(* Logix 5000 Rung export; software revision 16.04 *)

MODULES
   Local : vendor None type None code None
   MVI69E_AFC : vendor None type None code None
END_MODULES

TYPE AFCEMeterLinearLiquidArchive :   // Different Liquid Archive
STRUCT
   Write : AFCEMeterLinearLiquidArchiveWrite;
   Fetch : AFCEMeterLinearLiquidArchiveFetch;
END_STRUCT
END_TYPE

TYPE AFCESiteAlarms :   // Indicates if a meter has any alarms
STRUCT
   Meter1 : BOOL;   // Meter in alarm
   Meter2 : BOOL;   // Meter in alarm
   Meter3 : BOOL;   // Meter in alarm
   Meter4 : BOOL;   // Meter in alarm
   Meter5 : BOOL;   // Meter in alarm
   Meter6 : BOOL;   // Meter in alarm
   Meter7 : BOOL;   // Meter in alarm
   Meter8 : BOOL;   // Meter in alarm
   Meter9 : BOOL;   // Meter in alarm
   Meter10 : BOOL;   // Meter in alarm
   Meter11 : BOOL;   // Meter in alarm
   Meter12 : BOOL;   // Meter in alarm
   Meter13 : BOOL;   // Meter in alarm
   Meter14 : BOOL;   // Meter in alarm
   Meter15 : BOOL;   // Meter in alarm
   Meter16 : BOOL;   // Meter in alarm
END_STRUCT
END_TYPE

TYPE AFCEMeterLinearLiquid :   // Linear Liquid Meter
STRUCT
   Control : AFCEMeterControl;   // Meter Control
   Status : AFCEMeterStatus;   // Meter Status
   ProcessVariables : AFCEMeterLinearLiquidProcess;   // Input process variables to be transferred to the module
   Analysis : AFCEMeterAnalysis;   // Molar Analysis data to be transferred to the module (only for gas products with online gas chromatograph applications)
   Alarm : AFCEMeterLinearLiquidAlarm;   // Meter Alarms
   Archive : AFCEMeterLinearLiquidArchive;   // Archive
   Profile : AFCEMeterProfile;   // Module profile (meter type/product group) transfered from the module
   Calibration : AFCEMeterLinearLiquidCal;   // Calibration
   BackPlaneReturn : AFCEMeterLinearLiqBackPlaneReturn;
END_STRUCT
END_TYPE

TYPE AFCEFlag :   // Flags contains status information updated by ladder and also trigger bits for clock update
STRUCT
   AFCStopped : BOOL;   // Indicates that the module has sent a new input block to be processed by ladder - UPDATED BY LADDER
   AFCInputSequenceNum : INT;   // Meter number (0 -15) associated to blocks 1-16. Used to update "Profile" (meter type and product group.) UPDATED BY LADDER
END_STRUCT
END_TYPE

TYPE AFCEUtilBlockNonInterrupt :
STRUCT
   Now : BOOL;
   ModbusMasterCommand : BOOL;
   ModbusMasterResponse : BOOL;
   Archive : DINT;
   Prover : BOOL;
   PassThru : BOOL;
   Calibration : BOOL;
END_STRUCT
END_TYPE

TYPE AFCEMeterCalRequestActionType :
STRUCT
   ZeroShift : BOOL;   // Zero Shift
   SetZero : BOOL;   // Set Zero
   SetSpan : BOOL;   // Set Span
   SetMid1 : BOOL;   // Set Mid 1
   SetMid2 : BOOL;   // Set Mid 2
   SetMid3 : BOOL;   // Set Mid 3
END_STRUCT
END_TYPE

TYPE AFCEProveConfigEnable :   // Prove controls at enable
STRUCT
   MeterNumber : INT;   // Meter number requested (1-16)
   AutoAcceptProve : BOOL;   // Auto-accept the prove
   AutoContinueProve : BOOL;   // Auto-continue the prove
END_STRUCT
END_TYPE

TYPE AFCEModbusGateway :   // Modbus Gateway
STRUCT
   Command : AFCEModbusGatewayCommand[10];   // Modbus gateway commands - contains setup and modbus data
END_STRUCT
END_TYPE

TYPE AFCEMeterCalRequestActionValue :
STRUCT
   ZeroShift : AFCEMeterCalRequestValue;   // Zero Shift
   SetZero : AFCEMeterCalRequestValue;   // Set Zero
   SetSpan : AFCEMeterCalRequestValue;   // Set Span
   SetMid1 : AFCEMeterCalRequestValue;   // Set Mid 1
   SetMid2 : AFCEMeterCalRequestValue;   // Set Mid 2
   SetMid3 : AFCEMeterCalRequestValue;   // Set Mid 3
END_STRUCT
END_TYPE

TYPE AFCEMeterLinearLiqBackPlaneReturn :   // Linear Liquid Meter
STRUCT
   StandardDefault : AFCEMeterLinearLiquidStandardDataDflt;
   StandardRaw : INT[14];
   Extended : AFCEExtended;
END_STRUCT
END_TYPE

TYPE AFCEMeterLinearLiquidArchiveDflt :   // Default Configuration
STRUCT
   ClosingTimestamp : DINT;   // Closing Timestamp
   CumulativeActiveStreams : INT;
   CurrentActiveStream : SINT;
   MeterStatus : SINT;
   FlowingPeriod : DINT;
   PeriodDuration : DINT;
   AccumulatorTotalizer : DINT;
   AccumulatorResidue : REAL;
   MeterAlarms : DINT;
   PulseFrequency : REAL;
   Temperature : REAL;
   Pressure : REAL;
   Density : REAL;
   WaterContent : REAL;
   ReferenceDensity : REAL;
   Ctpl : REAL;
   KFactor : REAL;
   MeterFactor : REAL;
   InputPulseCount : DINT;
   ManPulseCountCurrent : DINT;
   MassNRAccumulatorCurrent : REAL;   // Non-resettable
   MassNRAccumulatorOpening : REAL;   // Non-resettable
   Available01 : INT;
   Available02 : INT;
   Available03 : INT;
   Available04 : INT;
   NetNRAccumulatorCurrent : REAL;   // Non-resettable
   NetNRAccumulatorOpening : REAL;   // Non-resettable
   GrossNRAccumulatorCurrent : REAL;   // Non-resettable
   GrossNRAccumulatorOpening : REAL;   // Non-resettable
   GrossStandardNRAccumulatorOpening : REAL;   // Non-resettable
   GrossStandardNRAccumulatorCurrent : REAL;   // Non-resettable
   WaterNRAccumulatorCurrent : REAL;   // Non-resettable
   WaterNRAccumulatorOpening : REAL;   // Non-resettable
   API2540VaporPressureAbsolute : REAL;   // Non-resettable
   Available05 : INT;
   Available06 : INT;
   UserSpecifiedFlowAverage1 : REAL;
   UserSpecifiedFlowAverage2 : REAL;
   UserSpecifiedFlowAverage3 : REAL;
END_STRUCT
END_TYPE

TYPE AFCEMeterAnalysisError :
STRUCT
   StreamOutOfRange : BOOL;   // Requested Stream Number Out of Range
   StreamNotConfigured : BOOL;   // Requested Stream Not Configured
END_STRUCT
END_TYPE

TYPE AFCEMeterLinearLiquidCalRequest :
STRUCT
   ProcessVariable : AFCEMeterLinearLiquidCalRequestProces;   // Process Variable
   ActionType : AFCEMeterCalRequestActionType;   // Action Type
   Value : AFCEMeterCalRequestActionValue;   // Value
   Count : DINT;   // Number of calibration requests
END_STRUCT
END_TYPE

TYPE AFCEMeterCalRequestValue :
STRUCT
   Applied : REAL;   // Applied
   Measured : REAL;   // Measured
END_STRUCT
END_TYPE

TYPE AFCEMeterLinearLiquidStandardDataDflt :   // EAFC Backplane Return Standard Data
STRUCT
   Meter_Alarms : DINT;   // Meter alarms
   NR_Acc_Net_Totalizer : DINT;   // Non-resettable accumulator, net, totalizer (m3)
   NR_Acc_Net_Residue : REAL;   // Non-resettable accumulator, net, residue (m3)
   FlowRate_Net : REAL;   // Flow rate, net (m3/h)
   NR_Acc_Gross_Totalizer : DINT;   // Non-resettable accumulator, gross / indicated, totalizer (m3)
   NR_Acc_GrossStandard_Totalizer : DINT;   // Non-resettable accumulator, gross standard, totalizer (m3)
   NR_Acc_Mass_Totalizer : DINT;   // Non-resettable accumulator, mass, totalizer (kg)
END_STRUCT
END_TYPE

TYPE AFCEModbusMasterDataType :   // Modbus master data type
STRUCT
   Bit : BOOL;   // bit type
   Word : BOOL;   // word type (16-bit)
   Long : BOOL;   // long integer (32-bit)
   LongRemote : BOOL;   // long integer (32-bit)
END_STRUCT
END_TYPE

TYPE AFCEUtil :   // Used for internal ladder logic usage. These values must not be changed by user application.
STRUCT
   Flags : AFCEFlag;   // Wallclock update commands
   CycleCounter : INT;   // Reflects current block ID calculated by ladder to be sent to the module
   Buffer : AFCEUtilBuffer;
   Block : AFCEUtilBlock;
END_STRUCT
END_TYPE

TYPE AFCEWallclock :
STRUCT
   GetAFCTime : BOOL;   // Get current AFC Time
   SetAFCTimeFromPLCTime : BOOL;   // Set AFC time from PLC time. Updates current AFC time
   EnableLocalDateTime : BOOL;   // Enable Local Date Time.
   AFCTime : AFCETime;   // Coordinated Universal Time. Updated by either getting or setting AFC time.
END_STRUCT
END_TYPE

TYPE AFCEProvePhaseBitmap :   // AFC prove phase bitmap
STRUCT
   NotSelected : BOOL;   // Not selected
   Active : BOOL;   // Active, not counting
   CountingPast1stSwitch : BOOL;   // Counting past 1st switch for Udir and forward leg for Bdir)
   Past2ndSwitchFwdLeg : BOOL;   // Past 2nd switch forward leg (bidirectional only)
   Past1stSwithRetLeg : BOOL;   // Past 1st switch return leg (bidirectional only)
   RunComplete : BOOL;   // Run complete. past 2nd switch.
END_STRUCT
END_TYPE

TYPE AFCEMeterLinearLiquidCalRequestProces :
STRUCT
   PulseFrequency : BOOL;   // Pulse Frequency
   Temperature : BOOL;   // Temperature
   Pressure : BOOL;   // Pressure
   Density : BOOL;   // Density
   WaterContent : BOOL;   // Water Content
END_STRUCT
END_TYPE

TYPE AFCEProveInputConfig :   // Prove input block results - prover configuration
STRUCT
   Type : INT;   // Prover type
   Options : INT;   // Prover options
   RunsPerProveTotal : INT;   // Total runs per prove
   RunsPerProveSelected : INT;   // Selected runs per prove
   MaxRunsBeforeAbort : INT;   // Max total runs before abort
   ShortPassesPerRun : INT;   // Short passes per run if bidir = 2 , else 0
END_STRUCT
END_TYPE

TYPE AFCEMeterCalResponse :
STRUCT
   Trigger : BOOL;   // Send Error Code and Values to module to be recorded
   ErrorCode : SINT;   // Error Code to send. 0-4 allowed. 0=No error. 1-4=User defined.
   Value : AFCEMeterCalRequestValue;   // Value to Send
   Count : DINT;   // Number of calibration responses
END_STRUCT
END_TYPE

TYPE AFCEMeterArchiveFetchError :
STRUCT
   ArchiveSelectionInvalid : BOOL;   // Archive File Selection Invalid
   AgeOutsideSize : BOOL;   // Age Outside Configured File Size
   ArchiveNeverWritten : BOOL;   // Age OK but Archive Record Never Written (new or reconfigured meter)
   Reserverd1 : BOOL;
   Reserverd2 : BOOL;
   Reserverd3 : BOOL;
   Reserverd4 : BOOL;
   Reserverd5 : BOOL;
   Reserverd6 : BOOL;
   Reserverd7 : BOOL;
   Reserverd8 : BOOL;
   Reserverd9 : BOOL;
   Reserverd10 : BOOL;
   Reserverd11 : BOOL;
   Reserverd12 : BOOL;
   Reserverd13 : BOOL;
END_STRUCT
END_TYPE

TYPE AFCEModbusGatewayCommand :   // Modbus Gateway Command
STRUCT
   Config : AFCEModbusGatewayConfig;   // Config data to be entered by the user.
   Trigger : BOOL;   // Trigger the Command, when cleared module has responded.
   Data : INT[200];   // Contains modbus data written to the module (write commands)
END_STRUCT
END_TYPE

TYPE AFCEProveConfigAccept :   // Prove controls at accept. If auto-accept is selected must be available at enable
STRUCT
   RequestedInterpolationPoint : INT;   // Requested interpolation point (0 nearest)
   ApplyMFChangeAllStreams : BOOL;   // Apply change in meter factor to all streams
   ApplyMFChangeCurve : BOOL;   // Apply change in meter factor to all curve points
   ApplyNewMF : BOOL;   // CApply new meter factor
END_STRUCT
END_TYPE

TYPE AFCEModbusMasterCommand :   // Modbus Master Command
STRUCT
   Config : AFCEModbusMasterConfig;   // Modbus Master Configuration
   ErrorCode : INT;   // Error Code associated to Modbus Master Command
   Pending : BOOL;   // Pending Modbus Master Command - waiting for Modbus Response
   ReturnedTransactionID : DINT;   // Changes to Config.TransactionID value when response has returned.
   Data : INT[100];   // Read or Write Data
END_STRUCT
END_TYPE

TYPE AFCEMeterStatusMeter :   // Meter Status
STRUCT
   Enabled : BOOL;   // Meter Enable Status, 1=enabled
   EnableAlarm : BOOL;   // If set either: 1. The meter is not configured. 2. The event log is full, the action was not performed.
END_STRUCT
END_TYPE

TYPE AFCEMeterLinearLiquidAlarmControl :   // Linear Liquid Process Alarms
STRUCT
   PulseFrequency : AFCEMeterProcessAlarm;   // Pulse Frequency Alarms
   Temperature : AFCEMeterProcessAlarm;   // Temperature Alarms
   Pressure : AFCEMeterProcessAlarm;   // Pressure Alarms
   Density : AFCEMeterProcessAlarm;   // Density Alarms
   WaterPercent : AFCEMeterProcessAlarm;   // Water Percent Alarms
   MeterPulses : AFCEMeterProcessAlarmFidelity;   // Meter Pulses Alarms
END_STRUCT
END_TYPE

TYPE AFCEMeterControl :   // Enable/Disable Meter and Streams
STRUCT
   Meter : AFCEMeterControlMeter;   // Control the Meter
   Stream : AFCEMeterControlStream;   // Control the Meter Streams
   ResetAccumulators : AFCEMeterSignals;   // Resets for meter accumulators
END_STRUCT
END_TYPE

TYPE AFCEProveSequencing :   // AFC prove sequencing tag for phase selection and ball positioning
STRUCT
   Phase : AFCEProvePhaseBitmap;   // AFC phase sequencing
   BallPositionReady : BOOL;   // Ball position: Ready (Udir & Bdir only; fwd leg Bdir)
   BallPositionSealed : BOOL;   // Ball position: Sealed (Udir & Bdir only; fwd leg Bdir)
   BallPositionReadyBwdLeg : BOOL;   // Ball position: Ready bwd leg (Bdir only)
   BallPositionSealedBwdLeg : BOOL;   // Ball position: Sealed bwd leg (Bdir only)
END_STRUCT
END_TYPE

TYPE AFCEMeterLinearLiquidProcess :   // Linear Liquid Process Variables
STRUCT
   PulseFrequency : REAL;   // Pulse frequency (Hz)
   Temperature : REAL;   // Temperature
   Pressure : REAL;   // Pressure
   Density : REAL;   // Density
   WaterPercent : REAL;   // Water (%)
   MeterPulses : DINT;   // Meter pulses
END_STRUCT
END_TYPE

TYPE AFCEUtilBlockInterrupt :
STRUCT
   Now : BOOL;
   ModbusGateway : DINT;
   EnableDisable : BOOL;
   Analysis : DINT;
END_STRUCT
END_TYPE

TYPE AFCEMeterLinearLiquidCal :   // Processor Mediated Calibration
STRUCT
   Request : AFCEMeterLinearLiquidCalRequest;   // Calibration Request from module
   Response : AFCEMeterCalResponse;   // Processor Response
END_STRUCT
END_TYPE

TYPE AFCEComponents :   // High precision gas component analysis (only supported version 2.07.000)
STRUCT
   C1 : REAL;   // Methane
   N2 : REAL;   // Nitrogen
   CO2 : REAL;   // Carbon Dioxide
   C2 : REAL;   // Ethane
   C3 : REAL;   // Propane
   H20 : REAL;   // Water
   H2S : REAL;   // Hydrogen Sulphide
   H2 : REAL;   // Hydrogen
   CO : REAL;   // Carbon Monoxide
   O2 : REAL;   // Oxygen
   IC4 : REAL;   // Iso-butane
   NC4 : REAL;   // Normal Butane
   IC5 : REAL;   // Iso-pentane
   NC5 : REAL;   // Normal-pentane
   C6 : REAL;   // Hexane
   C7 : REAL;   // Heptane
   C8 : REAL;   // Octane
   C9 : REAL;   // Nonane
   C10 : REAL;   // Decane
   He : REAL;   // Helium
   Ar : REAL;   // Argon
   NeoC5 : REAL;   // Not Used
   UxUser1 : REAL;   // Not Used
   UyUser2 : REAL;   // Not Used
   UxUser3 : REAL;   // Not Used
   UyUser4 : REAL;   // Not Used
   UxUser5 : REAL;   // Not Used
   UyUser6 : REAL;   // Not Used
   UxUser7 : REAL;   // Not Used
   UyUser8 : REAL;   // Not Used
   UxUser9 : REAL;   // Not Used
   UyUser10 : REAL;   // Not Used
END_STRUCT
END_TYPE

TYPE AFCEMeterStatus :   // Status
STRUCT
   Meter : AFCEMeterStatusMeter;   // Meter Status
   Stream : AFCEMeterStatusStream;   // Stream Status
END_STRUCT
END_TYPE

TYPE AFCEUtilBlock :
STRUCT
   ProcessInput : INT;
   InterruptPending : AFCEUtilBlockInterrupt;
   InterruptComplete : AFCEUtilBlockInterrupt;
   NonInterruptPending : AFCEUtilBlockNonInterrupt;
   NonInterruptComplete : AFCEUtilBlockNonInterrupt;
END_STRUCT
END_TYPE

TYPE AFCEModbusGatewayConfig :   // Modbus Ggateway Configuration
STRUCT
   Enable : BOOL;   // Set to 1 to enable modbus gateway command (0=disable)
   StartRegister : DINT;   // Start modbus address
   RegisterCount : INT;   // Word count (200 max)
   FunctionType : BOOL;   // 0 = read command, 1 = write command
   RegisterType : BOOL;   // 0 = holding register, 1 = input register
   SlaveType : BOOL;   // 0 = primary slave, 1 = virtual slave
END_STRUCT
END_TYPE

TYPE AFCEMeterControlMeter :   // Enable and Disable Meter
STRUCT
   Enable : BOOL;   // Enable the Meter
   Disable : BOOL;   // Disable the Meter
END_STRUCT
END_TYPE

TYPE AFCEMeterProfile :   // Meter configuration profile
STRUCT
   MeterType : BOOL;   // 0=Differential, 1=Linear
   ProductGroup : BOOL;   // 0=Gas, 1=Liquid
   PrimaryInput : BOOL;   // For differential, 0=Differential Pressure 1=Flow Rate. For Linear, 0=Pulse Count 1=Pulse Frequency
   AOIMismatch : BOOL;   // AOI Meter type does not match module for meter number
END_STRUCT
END_TYPE

TYPE AFCEModbusPassThru :   // AFC Modbus Pass-thru
STRUCT
   Enable : BOOL;   // Set to 1 to enable pass-thru functionality (requires AFC Manager setting)
   MessagePresent : BOOL;   // Message present in the response block
   GetMessage : BOOL;   // Get the pass-thru message. When the bit is cleared the message has been transferred to the PLC.
   FunctionBitWrite : BOOL;   // Function bit write
   OverflowError : BOOL;   // Overflow error flag
   ModbusAddress : INT;   // Destination modbus address
   RegisterCount : INT;   // Number of elements associated to command
   ReadDataWord : INT[125];   // Contains received data for word commands
   ReadDataBit : AFCEModbusPassThruBitData;   // Contains received data for bit commands
END_STRUCT
END_TYPE

TYPE AFCEUtilBuffer :   // Buffer
STRUCT
   Input : INT[248];   // Input buffer contains the complete block to be copied from the module
   Output : INT[247];   // Output buffer contains data the complete block to be copied to the module
   Process : INT[180];
   ArchiveDay : INT[98];
   ArchiveHour : INT[98];
   Prove : INT[26];
   Analysis : INT[198];
   MeterEnableDisable : INT[4];
   StreamEnable : INT[36];
   StreamDisable : INT[36];
   StreamSelect : INT[24];
   MeterSignals : INT[24];
   Calibration : INT[36];
END_STRUCT
END_TYPE

TYPE AFCEProveStatus :   // Status of the prove (returned from the module to the processor)
STRUCT
   ProveAccepted : BOOL;   // Prove was accepted
   MeterFactorApplied : BOOL;   // Meter factor was applied
   MFAppliedToCurve : BOOL;   // Meter factor was applied to all points in the curve
   MFAppliedToStreams : BOOL;   // Meter factor was applied to all streams
   ProveRejectedByCommand : BOOL;   // Prove was rejected by command
   ProveRejectedNoRuns : BOOL;   // Prove was rejected - empty prove (no runs)
   ProveRejectedDivideBy0 : BOOL;   // Prove was rejected - divide by 0
   ProveEnabled : BOOL;   // Prove is enabled
   ProvingRunInProgress : BOOL;   // Proving run is in progress
   ProveRejectedAbort : BOOL;   // Prove rejected: abort
   ProvePaused : BOOL;   // Prove is paused
   RunCancelled : BOOL;   // Run Is cancelled
   RunTimedOut : BOOL;   // Run timed out
END_STRUCT
END_TYPE

TYPE AFCEMeterStatusStreamAlarm :   // Stream Alarms
STRUCT
   StreamOutOfRange : BOOL;   // Requested Stream Number Out of Range
   StreamNotConfigured : BOOL;   // Requested Stream not Configured
   StreamNotEnabled : BOOL;   // Requested Stream not Enabled
   EventLogFull : BOOL;   // Event Log Full, Action not Performed
END_STRUCT
END_TYPE

TYPE AFCEProveConfig :   // Controls (configuration settings) associated to the prover
STRUCT
   Enable : AFCEProveConfigEnable;   // Controls at enable
   Accept : AFCEProveConfigAccept;   // Controls at accept
END_STRUCT
END_TYPE

TYPE AFCESiteStatus :   // Site status bits - contains general information about the module - not meter specific
STRUCT
   AFCActive : BOOL;   // AFC active
   ChecksumAlarms : BOOL;   // Checkum alarm active
   Reserved2 : BOOL;
   Reserved3 : BOOL;
   PLCHalted : BOOL;   // PLC in program mode or missing
   CfgChanged : BOOL;   // Configuration changed
   Powerup : BOOL;   // Module powered up
   ColdStart : BOOL;   // Module performed cold start (BBRAM initialized)
   ModbusMasterPending : BOOL;   // Modbus Master Poll Pending
   ModbusMasterComplete : BOOL;   // Modbus Master Poll Complete
   ModbusPassThruPending : BOOL;   // Modbus Pass-thru Input Pending
   CalibrationRequest : BOOL;   // Calibration request from module
   ProverEnabled : BOOL;   // Prover Enabled
   Reserved13 : BOOL;
   Reserved14 : BOOL;
   Reserved15 : BOOL;
END_STRUCT
END_TYPE

TYPE AFCEModbusMaster :   // Modbus Master. Port 3 must be configured as modbus master through AFC Manager to use this feature.
STRUCT
   Enable : BOOL;   // Enable the modbus master funcionality
   CommandIndex : INT;   // Selects which command index will be executed
   Command : AFCEModbusMasterCommand[10];   // Each command contains a specific modbus request to be sent out of the port
END_STRUCT
END_TYPE

TYPE AFCEProveProcess :   // Prove process output from processor to the module
STRUCT
   Sequencing : AFCEProveSequencing;   // Prover sequencing
   Temperature : REAL;   // Temperature for Single Probe provers. And Inlet Temperature for Dual Probe Provers.
   OutletTemperature : REAL;   // Outlet Temperature for Provers with Dual Probes.
   SwitchBarTemperature : REAL;   // Switch bar temperature
   Pressure : REAL;   // Pressure for Single Probe provers. And Inlet Pressure for Dual Probe Provers.
   OutletPressure : REAL;   // Outlet Pressure for Provers with Dual Probes.
   ProverDensity : REAL;   // Prover density
END_STRUCT
END_TYPE

TYPE AFCEExtended :
STRUCT
   Trigger : BOOL;
   Data : AFCEExtendedData;
END_STRUCT
END_TYPE

TYPE AFCEMeterSignals :   // Meter trigger accumulator and archive resets
STRUCT
   ResetAccumulator1 : BOOL;   // Set to 1 to reset resettable accumulator 1
   ResetAccumulator2 : BOOL;   // Set to 1 to reset resettable accumulator 2
   ResetAccumulator3 : BOOL;   // Set to 1 to reset resettable accumulator 3
   ResetAccumulator4 : BOOL;   // Set to 1 to reset resettable accumulator 4
END_STRUCT
END_TYPE

TYPE AFCEMeterProcessAlarm :   // Process Alarms
STRUCT
   SetGeneralFail : BOOL;   // Set to indicate General Failure of the Transmitter
   StaleData : BOOL;   // Clear to Indicate new process input data
   SetLowThreshold : BOOL;   // Set to indicate Lower Range Limit Exceeded
   SetHighThreshold : BOOL;   // Set to indicate Upper Range Limit Exceeded
   SetAutoClearStaleData : BOOL;   // Set to automatically clear stale data
END_STRUCT
END_TYPE

TYPE AFCETime :   // AFC time format used for wallclock update.
STRUCT
   Year : DINT;   // Year
   Month : DINT;   // Month
   Day : DINT;   // Day
   Hour : DINT;   // Hour
   Minute : DINT;   // Minute
   second : DINT;   // Seconds
END_STRUCT
END_TYPE

TYPE AFCEModbusMasterSwap :   // Modbus master swap words/ swap bytes
STRUCT
   SwapWords : BOOL;   // Swap words
   SwapBytes : BOOL;   // Swap bytes
END_STRUCT
END_TYPE

TYPE AFCEMeterControlStream :
STRUCT
   Selected : SINT;   // Stream to Enable or Disable and/or make active.
   EnableSelected : BOOL;   // Enable the Selected Stream
   DisableSelected : BOOL;   // Disable the Selected Stream
   SetSelectedToActive : BOOL;   // Set Selected to Active Stream
END_STRUCT
END_TYPE

TYPE AFCEProvePulseCount :   // Values to be supplied at the end of the pass/run
STRUCT
   Meter : DINT;   // Meter pulse count
   MasterMeter : DINT;   // Master meter pulse count
END_STRUCT
END_TYPE

TYPE AFCEMeterLinearLiquidArchiveFetchT :   // Fetch Archive
STRUCT
   Trigger : BOOL;   // Trigger Archive Fetch
   Age : INT;   // 0 = Current Archive
   Error : AFCEMeterArchiveFetchError;   // Archive Fetch Error
   Default : AFCEMeterLinearLiquidArchiveDflt;   // Default Archive
   Raw : INT[100];   // Raw Archive
END_STRUCT
END_TYPE

TYPE AFCEMeterStatusStream :
STRUCT
   Active : INT;   // Current Active Stream
   Enabled : AFCEMeterStatusStreamEnabled;   // Enabled Streams
   Configured : AFCEMeterStatusStreamEnabled;   // Configured Streams
   EnableAlarm : AFCEMeterStatusStreamAlarm;   // Enable Alarms
END_STRUCT
END_TYPE

TYPE AFCEExtendedData :
STRUCT
   Raw : INT[64];
END_STRUCT
END_TYPE

TYPE AFCEMeterLinearLiquidArchiveWrite :   // Write Archive
STRUCT
   Daily : BOOL;   // Set to 1 to write daily archive
   Hourly : BOOL;   // Set to 1 to write hourly archive
END_STRUCT
END_TYPE

TYPE AFCEModbusPassThruBitData :   // AFC Modbus Pass-thru Bit Data
STRUCT
   Data : BOOL[2016];   // Contains received data for bit commands
END_STRUCT
END_TYPE

TYPE AFCEModbusMasterConfig :   // Modbus master command settings
STRUCT
   Enable : BOOL;   // Set to 1 to enable command (0=disable)
   FunctionType : BOOL;   // Set to 1 to select write command (0=read command)
   RegisterBank : BOOL;   // Set to 1 to select input register (0=holding register)
   DataType : AFCEModbusMasterDataType;   // Select data type format
   SwapOption : AFCEModbusMasterSwap;   // Select byte and word swap (1 = swap, 0 = no swap)
   TypeSwap : INT;   // This value is calculated by ladder logic and must not be modified by user
   SlaveAddress : INT;   // Modbus slave address of remote device
   ModbusAddress : INT;   // Modbus data address on remote slave
   ElementCount : INT;   // Number of data elements (125 words)
   TransactionID : INT;   // Transaction ID. This value is returned to the ReturnedTransaction ID when the response has been received.
END_STRUCT
END_TYPE

TYPE AFCEMeterProcessAlarmFidelity :   // Process Alarms
STRUCT
   SetGeneralFail : BOOL;   // Set to indicate General Failure of the Transmitter
   StaleData : BOOL;   // Clear to Indicate new process input data
   Reserved : BOOL;   // Reserved
   SetPulseFidelityAlarm : BOOL;   // Set to indicate Pulse Fidelity Alarm
   SetAutoClearStaleData : BOOL;   // Set to automatically clear stale data
END_STRUCT
END_TYPE

TYPE AFCEModuleDef :   // Main user defined data type
STRUCT
   ModbusGateway : AFCEModbusGateway;   // Reads and write data between processor and module modbus table
   ModbusMaster : AFCEModbusMaster;   // Setup modbus master commands to be sent to remote slaves (through Port 3)
   ModbusPassThru : AFCEModbusPassThru;   // Modbus pass-thru data
   SiteStatus : AFCESiteStatus;   // Site status
   MeterAlarms : AFCESiteAlarms;   // Meter Alarms
   Prove : AFCEProve;   // Prover
   Wallclock : AFCEWallclock;   // Set clock and get clock information
   Firmware : AFCEFirmwareVersion;   // Firmware information
   Util : AFCEUtil;   // Used by ladder logic
END_STRUCT
END_TYPE

TYPE AFCEMeterAnalysis :   // Meter analysis components. Allows the processor to update molar analysis for low precision and high precision streams.
STRUCT
   Trigger : BOOL;   // Set to 1 to Send Updated Component Data to the Module
   Stream : INT;   // Stream for Analysis. Select 0 for current active stream.
   Error : AFCEMeterAnalysisError;   // Analysis Error
   Components : AFCEComponents;   // High precision gas components (floating point per component). Only supported for firmware version 2.07.000 or later
END_STRUCT
END_TYPE

TYPE AFCEProveSignals :   // Contains the proving signals that will trigger specific tasks from the module
STRUCT
   EnableProve : BOOL;   // Enables the prove
   AcceptProve : BOOL;   // Accepts the prove
   RejectProve : BOOL;   // Reject the prove
   RunStart : BOOL;   // Starts the run
   RunComplete : BOOL;   // Flags that the run is complete
   RunCancel : BOOL;   // Cancels the run
   RunDelete : BOOL;   // Deletes the run
   PassComplete : BOOL;   // Flag that the pass is complete
   PauseProve : BOOL;   // Pauses the Proving Process
   AbortProve : BOOL;   // Aborts the prove
END_STRUCT
END_TYPE

TYPE AFCEFirmwareVersion :
STRUCT
   Major : SINT;   // Major Version number
   Minor : SINT;   // Minor Version number
   Revision : INT;   // Revision
END_STRUCT
END_TYPE

TYPE AFCEMeterLinearLiquidArchiveFetch :
STRUCT
   Daily : AFCEMeterLinearLiquidArchiveFetchT;
   Hourly : AFCEMeterLinearLiquidArchiveFetchT;
END_STRUCT
END_TYPE

TYPE AFCEProveRunResults :   // Run results of the prove. Copied from the module to the pocessor
STRUCT
   CountAttempted : INT;   // Run count attempted
   CountCompleted : INT;   // Run count completed
   CountSelected : INT;   // Run count selected
   RunsSelected : INT;   // Bit Mapped Runs selected for calculations from completed runs
   NewMeterFactor : REAL;   // New meter factor
   ChangeInMeterFactor : REAL;   // Change in meter factor
END_STRUCT
END_TYPE

TYPE AFCEMeterStatusStreamEnabled :   // Stream Status 1 = Enabled
STRUCT
   Stream1 : BOOL;
   Stream2 : BOOL;
   Stream3 : BOOL;
   Stream4 : BOOL;
   Stream5 : BOOL;
   Stream6 : BOOL;
   Stream7 : BOOL;
   Stream8 : BOOL;
   Stream9 : BOOL;
   Stream10 : BOOL;
   Stream11 : BOOL;
   Stream12 : BOOL;
   Stream13 : BOOL;
   Stream14 : BOOL;
   Stream15 : BOOL;
   Stream16 : BOOL;
END_STRUCT
END_TYPE

TYPE AFCEMeterLinearLiquidAlarm :
STRUCT
   Control : AFCEMeterLinearLiquidAlarmControl;   // Alarm Control
END_STRUCT
END_TYPE

TYPE AFCEProve :   // Prove
STRUCT
   Process : AFCEProveProcess;   // Process Variables
   Signals : AFCEProveSignals;   // AFC Prove Signals (triggers the proving update)
   Config : AFCEProveConfig;   // AFC Prove Control (configuration settings)
   PulseCounts : AFCEProvePulseCount;   // Pulse counts to be updated at the end of the run/pass
   ConfigInput : AFCEProveInputConfig;   // AFC prover input configuration
   Status : AFCEProveStatus;   // AFC prover status
   ErrorCode : INT;   // Prove error code
   ProveControlsEcho : INT;   // AFC module Echos the state of the Prove Controls
   RequestedMeterEcho : INT;   // AFC module Echos the Meter number requested
   RequestedCurvePointEcho : INT;   // AFC module Echos the requested Curve Point
   RunResults : AFCEProveRunResults;   // Prove and run results
   ProveEnabled : BOOL;   // ON if prove is enabled. This flag is coped from inputbuffer[247]
END_STRUCT
END_TYPE

ADD_ON_INSTRUCTION AOI69EAFCMeterLinearLiquid   (* revision 1.5, vendor ProSoft Technology Inc., ExecutePrescan *)
// Add-On instruction for the MVI69E-AFC.
// Linear Liquid Meter.
// Revision note:
// Updated  BackplaneReturn Tag name from ProcessInputs to Standard
// and ComponentAnalysis to Extended
// Help:
// Compatible with version 4.04 of MVI69E-AFC firmware or higher.
// v1.1: Comp Analysis Return fix
// v1.2: Addition of default process input backplane return data mapping.
// v1.3: Changed Prescan FLL instruction length from 240 words to 180 for proccess inputs. This stopped mismatch issue.
// v1.3: Made correlation changes between the Module Archive Default UDTs and the AOI Archive Default UDTs.
// v1.4: Made changes to the ModbusGatewayConfig UDT StartRegister Tag Data Type from INT to DINT.
// v1.5: Updated Tags names AFCMeterXXYYYYYY.BackPlaneReturn.ProcessInputs to
// AFCMeterXXYYYYYY.BackPlaneReturn.Standard and
// AFCMeterXXYYYYYY.BackPlaneReturn.ComponentAnalysis
//  to AFCMeterXXYYYYYY.BackPlaneReturn.Extended.
VAR_IN_OUT
   ConnectionInput : INT[248]; {required}
   AFC : AFCEModuleDef; {required}
   AFCMeter : AFCEMeterLinearLiquid; {required}
END_VAR
VAR_INPUT
   MeterNumber : SINT; {required}   // Meter Number Set to a number between 1 and 12
END_VAR
VAR
   StreamSelectedShift : DINT;
   StreamSelectBuffer : INT;
   EnabledStatusBuffer : INT;
   StreamSelectBlockID : DINT;
   StreamNumberShift : DINT;
   StreamErrorBuffer : DINT;
   StreamEnableBlockID : DINT;
   StreamEnableBitPosition : DINT;
   StreamDisableBlockID : DINT;
   ResetOnce : BOOL;
   ProfileBuffer : SINT[2];
   ProcessInputBlockID : DINT;
   AnalysisGroupBitPosition : INT;
   AnalysisErrorBuffer : INT;
   ProcessAlarmShifter : DINT;
   ProcessAlarmHolder : DINT;
   ProcessAlarmBuffer : DINT;
   MeterSignaltBlockID : DINT;
   MeterNumberShift : DINT;
   MeterNumberBitPostition : DINT;
   Inputbuffer : INT[248];
   CalibrationMeterNumberBuffer : DINT;
   CalibrationMediationPending : BOOL;
   CalibrationInputScalingIndex : DINT;
   CalibrationHandleBuffer : DINT;
   ArchiveStream : DINT;
   ArchiveMeterStatusRaw : DINT;
   ArchiveMeterStatusActiveStream : DINT;
   ArchiveCompleteBitCheck : DINT;
   ArchiveBlockID : DINT;
   AnalysisGroupShift : DINT;
   AnalysisCompleteBitCheck : DINT;
   AnalysisBufferOffset : DINT;
   AFCStopped : BOOL;
   AFCInputDataAvailable : BOOL;
   AnalysisBlockID : DINT;
END_VAR

ROUTINE Logic   (* ladder *)
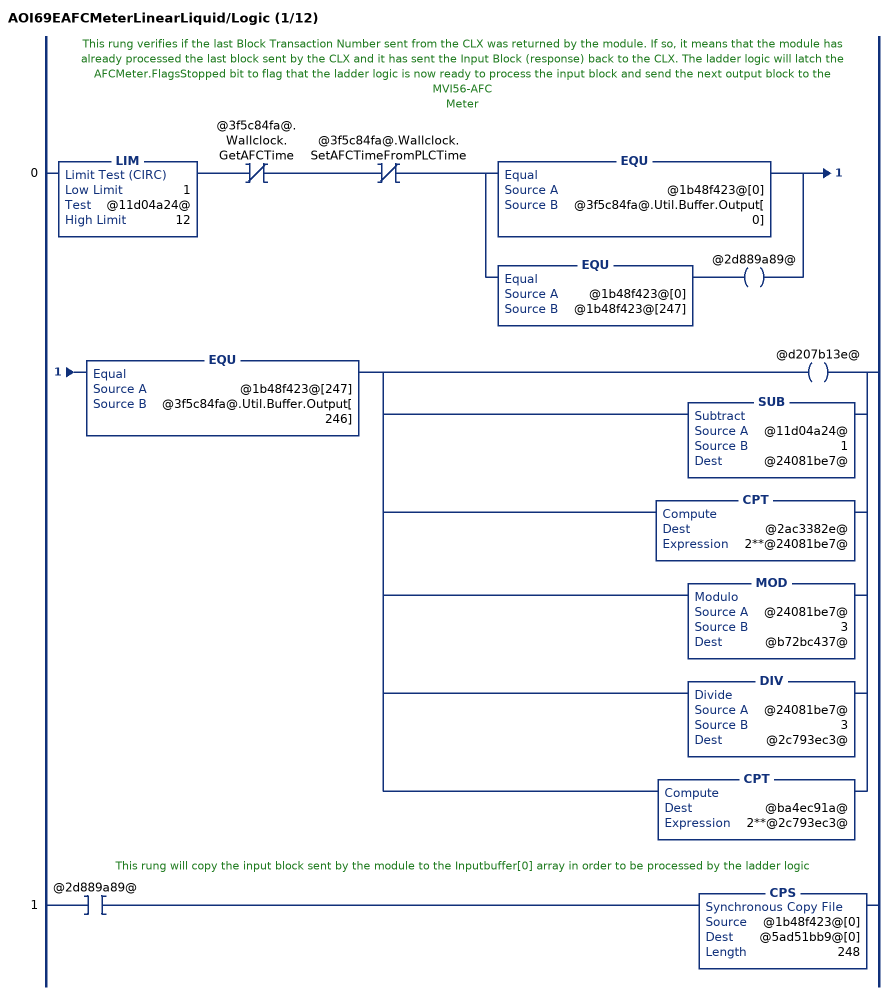
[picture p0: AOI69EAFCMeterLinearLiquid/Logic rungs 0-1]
   // This rung verifies if the last Block Transaction Number sent from the CLX was returned by the module. If so, it means that the module has already processed the last block sent by the CLX and it has sent the Input Block (response) back to the CLX. The ladder logic will latch the AFCMeter.FlagsStopped bit to flag that the ladder logic is now ready to process the input block and send the next output block to the MVI56-AFC
   // Meter
   0: LIM(1,@11d04a24@,12)XIO(@3f5c84fa@.Wallclock.GetAFCTime)XIO(@3f5c84fa@.Wallclock.SetAFCTimeFromPLCTime)[EQU(@1b48f423@[0],@3f5c84fa@.Util.Buffer.Output[0]) ,EQU(@1b48f423@[0],@1b48f423@[247]) OTE(@2d889a89@) ]EQU(@1b48f423@[247],@3f5c84fa@.Util.Buffer.Output[246])[OTE(@d207b13e@) ,SUB(@11d04a24@,1,@24081be7@) ,CPT(@2ac3382e@,2**@24081be7@) ,MOD(@24081be7@,3,@b72bc437@) ,DIV(@24081be7@,3,@2c793ec3@) ,CPT(@ba4ec91a@,2**@2c793ec3@) ];
   // This rung will copy the input block sent by the module to the Inputbuffer[0] array in order to be processed by the ladder logic
   1: XIC(@2d889a89@)CPS(@1b48f423@[0],@5ad51bb9@[0],248);
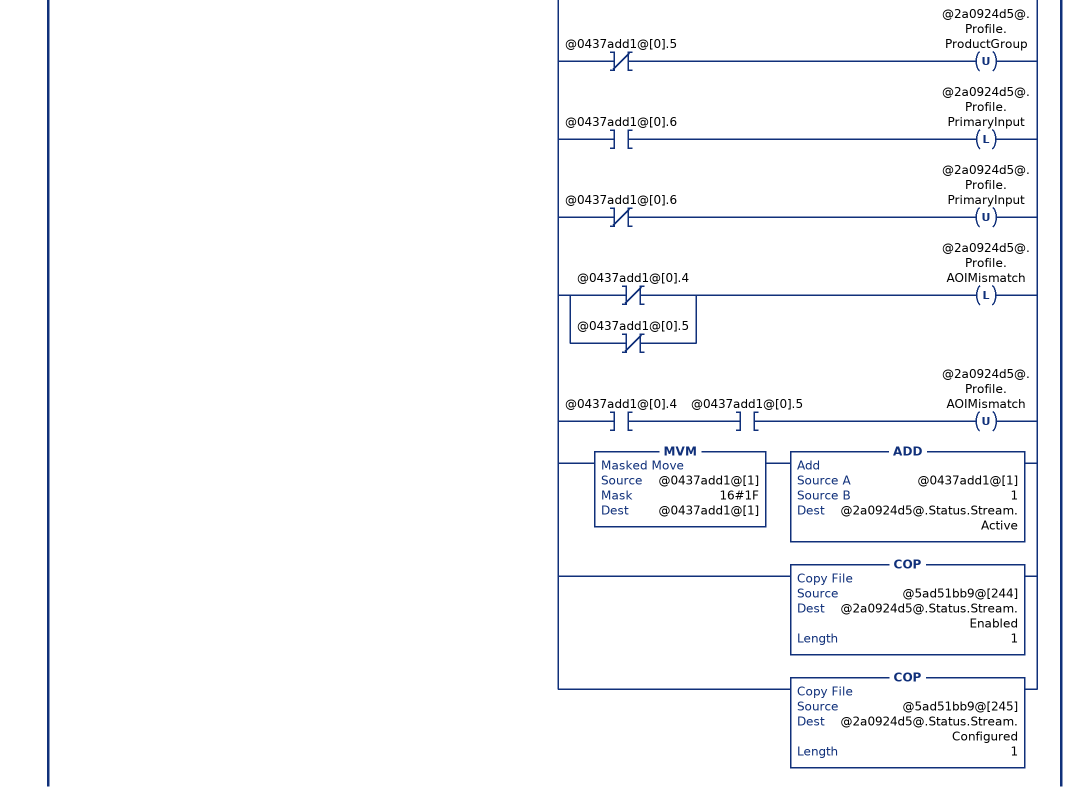
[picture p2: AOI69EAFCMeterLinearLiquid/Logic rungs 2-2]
   // Read process input backplane return and
   // meter profile (when block ID matches meter number).
   2: XIC(@2d889a89@)LIM(1,@5ad51bb9@[0],12)[COP(@5ad51bb9@[3+@24081be7@*15],@2a0924d5@.BackPlaneReturn.StandardRaw[0],14) ,COP(@2a0924d5@.BackPlaneReturn.StandardRaw[0],@2a0924d5@.BackPlaneReturn.StandardDefault,1) ,COP(@5ad51bb9@[246],@3f5c84fa@.SiteStatus,1) ,EQU(@5ad51bb9@[0],@11d04a24@) [COP(@5ad51bb9@[243],@0437add1@[0],2) ,[XIC(@0437add1@[0].0) OTL(@2a0924d5@.Status.Meter.EnableAlarm) ,XIO(@0437add1@[0].0) OTU(@2a0924d5@.Status.Meter.EnableAlarm) ] ,[XIC(@0437add1@[0].1) OTL(@2a0924d5@.Status.Meter.Enabled) ,XIO(@0437add1@[0].1) OTU(@2a0924d5@.Status.Meter.Enabled) ] ,[[XIC(@0437add1@[0].4) OTL(@2a0924d5@.Profile.MeterType) ,XIO(@0437add1@[0].4) OTU(@2a0924d5@.Profile.MeterType) ] ,[XIC(@0437add1@[0].5) OTL(@2a0924d5@.Profile.ProductGroup) ,XIO(@0437add1@[0].5) OTU(@2a0924d5@.Profile.ProductGroup) ] ,[XIC(@0437add1@[0].6) OTL(@2a0924d5@.Profile.PrimaryInput) ,XIO(@0437add1@[0].6) OTU(@2a0924d5@.Profile.PrimaryInput) ] ] ,[[XIO(@0437add1@[0].4) ,XIO(@0437add1@[0].5) ] OTL(@2a0924d5@.Profile.AOIMismatch) ,XIC(@0437add1@[0].4) XIC(@0437add1@[0].5) OTU(@2a0924d5@.Profile.AOIMismatch) ] ,MVM(@0437add1@[1],16#1F,@0437add1@[1]) ADD(@0437add1@[1],1,@2a0924d5@.Status.Stream.Active) ,COP(@5ad51bb9@[244],@2a0924d5@.Status.Stream.Enabled,1) ,COP(@5ad51bb9@[245],@2a0924d5@.Status.Stream.Configured,1) ] ];
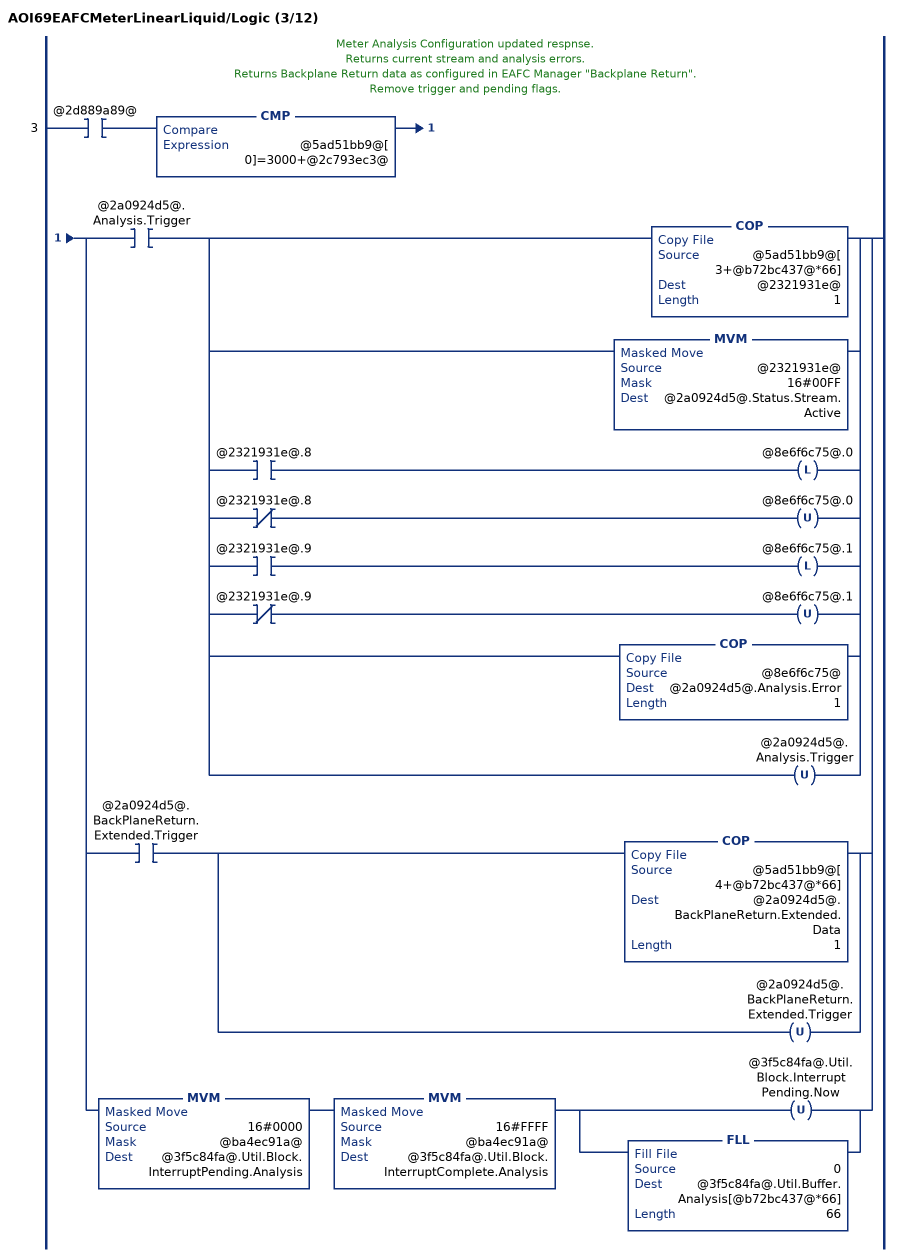
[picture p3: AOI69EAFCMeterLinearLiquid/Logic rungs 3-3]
   // Meter Analysis Configuration updated respnse.
   // Returns current stream and analysis errors.
   // Returns Backplane Return data as configured in EAFC Manager "Backplane Return".
   // Remove trigger and pending flags.
   3: XIC(@2d889a89@)CMP(@5ad51bb9@[0]=3000+@2c793ec3@)[XIC(@2a0924d5@.Analysis.Trigger) [COP(@5ad51bb9@[3+@b72bc437@*66],@2321931e@,1) ,MVM(@2321931e@,16#00FF,@2a0924d5@.Status.Stream.Active) ,[XIC(@2321931e@.8) OTL(@8e6f6c75@.0) ,XIO(@2321931e@.8) OTU(@8e6f6c75@.0) ] ,[XIC(@2321931e@.9) OTL(@8e6f6c75@.1) ,XIO(@2321931e@.9) OTU(@8e6f6c75@.1) ] ,COP(@8e6f6c75@,@2a0924d5@.Analysis.Error,1) ,OTU(@2a0924d5@.Analysis.Trigger) ] ,XIC(@2a0924d5@.BackPlaneReturn.Extended.Trigger) [COP(@5ad51bb9@[4+@b72bc437@*66],@2a0924d5@.BackPlaneReturn.Extended.Data,1) ,OTU(@2a0924d5@.BackPlaneReturn.Extended.Trigger) ] ,MVM(16#0000,@ba4ec91a@,@3f5c84fa@.Util.Block.InterruptPending.Analysis) MVM(16#FFFF,@ba4ec91a@,@3f5c84fa@.Util.Block.InterruptComplete.Analysis) [OTU(@3f5c84fa@.Util.Block.InterruptPending.Now) ,FLL(0,@3f5c84fa@.Util.Buffer.Analysis[@b72bc437@*66],66) ] ];
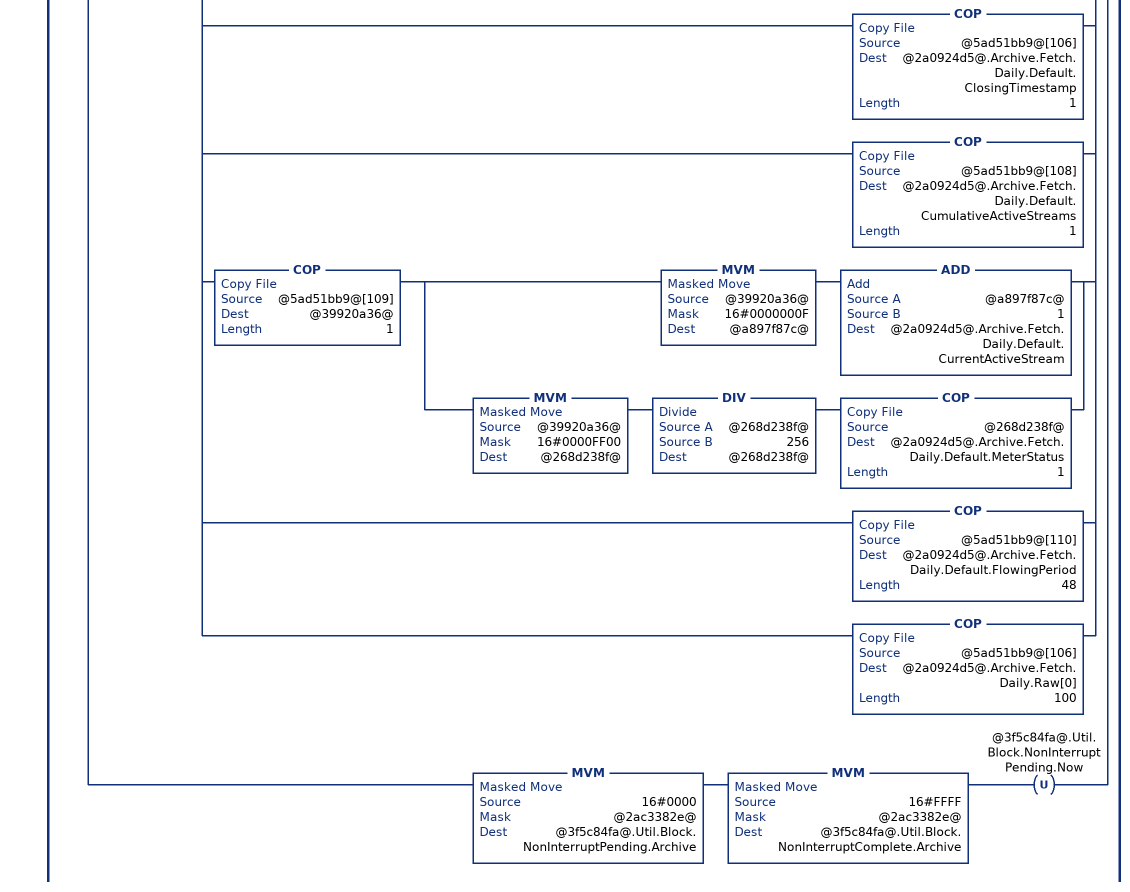
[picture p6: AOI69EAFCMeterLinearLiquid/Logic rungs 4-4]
   // Archive Fetch to default and raw UDT's.
   // Get archive alarms.
   // Remove trigger and pending flags.
   4: XIC(@2d889a89@)CMP(@5ad51bb9@[0]=6000+@24081be7@)[XIC(@2a0924d5@.Archive.Fetch.Hourly.Trigger) [OTU(@2a0924d5@.Archive.Fetch.Hourly.Trigger) ,[[XIC(@5ad51bb9@[3].0) OTL(@2a0924d5@.Archive.Fetch.Hourly.Error.ArchiveSelectionInvalid) ,XIO(@5ad51bb9@[3].0) OTU(@2a0924d5@.Archive.Fetch.Hourly.Error.ArchiveSelectionInvalid) ] ,[XIC(@5ad51bb9@[3].1) OTL(@2a0924d5@.Archive.Fetch.Hourly.Error.AgeOutsideSize) ,XIO(@5ad51bb9@[3].1) OTU(@2a0924d5@.Archive.Fetch.Hourly.Error.AgeOutsideSize) ] ,[XIC(@5ad51bb9@[3].2) OTL(@2a0924d5@.Archive.Fetch.Hourly.Error.ArchiveNeverWritten) ,XIO(@5ad51bb9@[3].2) OTU(@2a0924d5@.Archive.Fetch.Hourly.Error.ArchiveNeverWritten) ] ] ,COP(@5ad51bb9@[4],@2a0924d5@.Archive.Fetch.Hourly.Default.ClosingTimestamp,1) ,COP(@5ad51bb9@[6],@2a0924d5@.Archive.Fetch.Hourly.Default.CumulativeActiveStreams,1) ,COP(@5ad51bb9@[7],@39920a36@,1) [MVM(@39920a36@,16#0000000F,@a897f87c@) ADD(@a897f87c@,1,@2a0924d5@.Archive.Fetch.Hourly.Default.CurrentActiveStream) ,MVM(@39920a36@,16#0000FF00,@268d238f@) DIV(@268d238f@,256,@268d238f@) COP(@268d238f@,@2a0924d5@.Archive.Fetch.Hourly.Default.MeterStatus,1) ] ,COP(@5ad51bb9@[8],@2a0924d5@.Archive.Fetch.Hourly.Default.FlowingPeriod,48) ,COP(@5ad51bb9@[4],@2a0924d5@.Archive.Fetch.Hourly.Raw[0],100) ] ,XIC(@2a0924d5@.Archive.Fetch.Daily.Trigger) [OTU(@2a0924d5@.Archive.Fetch.Daily.Trigger) ,[[XIC(@5ad51bb9@[105].0) OTL(@2a0924d5@.Archive.Fetch.Daily.Error.ArchiveSelectionInvalid) ,XIO(@5ad51bb9@[105].0) OTU(@2a0924d5@.Archive.Fetch.Daily.Error.ArchiveSelectionInvalid) ] ,[XIC(@5ad51bb9@[105].1) OTL(@2a0924d5@.Archive.Fetch.Daily.Error.AgeOutsideSize) ,XIO(@5ad51bb9@[105].1) OTU(@2a0924d5@.Archive.Fetch.Daily.Error.AgeOutsideSize) ] ,[XIC(@5ad51bb9@[105].2) OTL(@2a0924d5@.Archive.Fetch.Daily.Error.ArchiveNeverWritten) ,XIO(@5ad51bb9@[105].2) OTU(@2a0924d5@.Archive.Fetch.Daily.Error.ArchiveNeverWritten) ] ] ,COP(@5ad51bb9@[106],@2a0924d5@.Archive.Fetch.Daily.Default.ClosingTimestamp,1) ,COP(@5ad51bb9@[108],@2a0924d5@.Archive.Fetch.Daily.Default.CumulativeActiveStreams,1) ,COP(@5ad51bb9@[109],@39920a36@,1) [MVM(@39920a36@,16#0000000F,@a897f87c@) ADD(@a897f87c@,1,@2a0924d5@.Archive.Fetch.Daily.Default.CurrentActiveStream) ,MVM(@39920a36@,16#0000FF00,@268d238f@) DIV(@268d238f@,256,@268d238f@) COP(@268d238f@,@2a0924d5@.Archive.Fetch.Daily.Default.MeterStatus,1) ] ,COP(@5ad51bb9@[110],@2a0924d5@.Archive.Fetch.Daily.Default.FlowingPeriod,48) ,COP(@5ad51bb9@[106],@2a0924d5@.Archive.Fetch.Daily.Raw[0],100) ] ,MVM(16#0000,@2ac3382e@,@3f5c84fa@.Util.Block.NonInterruptPending.Archive) MVM(16#FFFF,@2ac3382e@,@3f5c84fa@.Util.Block.NonInterruptComplete.Archive) OTU(@3f5c84fa@.Util.Block.NonInterruptPending.Now) ];
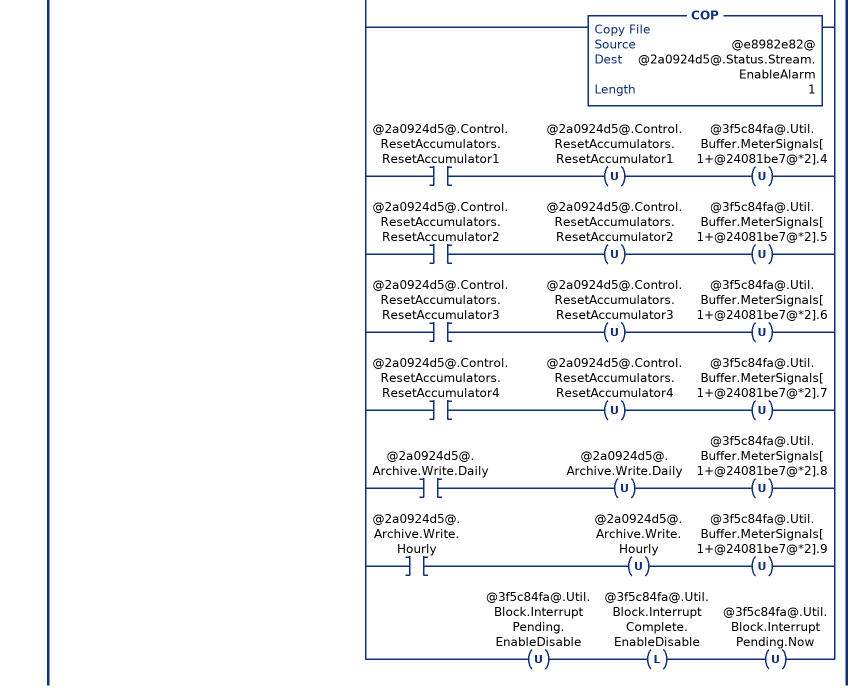
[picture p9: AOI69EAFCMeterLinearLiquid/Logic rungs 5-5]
   // Meter status and stream status.
   // Remove trigger and pending flags.
   5: XIC(@2d889a89@)EQU(@5ad51bb9@[0],7000)[[MVM(@5ad51bb9@[3],@2ac3382e@,@778da0e9@) ,[NEQ(@778da0e9@,0) OTL(@2a0924d5@.Status.Meter.Enabled) ,EQU(@778da0e9@,0) OTU(@2a0924d5@.Status.Meter.Enabled) ] ,OTU(@2a0924d5@.Control.Meter.Enable) MVM(16#0000,@2ac3382e@,@3f5c84fa@.Util.Buffer.MeterEnableDisable[1]) ,OTU(@2a0924d5@.Control.Meter.Disable) MVM(16#0000,@2ac3382e@,@3f5c84fa@.Util.Buffer.MeterEnableDisable[3]) ] ,[XIC(@2a0924d5@.Control.Stream.EnableSelected) [COP(@5ad51bb9@[7+@24081be7@*3],@2a0924d5@.Status.Stream.Enabled,1) ,COP(@5ad51bb9@[8+@24081be7@*3],@2a0924d5@.Status.Stream.Configured,1) ,OTU(@2a0924d5@.Control.Stream.EnableSelected) OTU(@2a0924d5@.Control.Stream.DisableSelected) ] ,XIC(@2a0924d5@.Control.Stream.DisableSelected) [COP(@5ad51bb9@[55+@24081be7@*3],@2a0924d5@.Status.Stream.Enabled,1) ,COP(@5ad51bb9@[56+@24081be7@*3],@2a0924d5@.Status.Stream.Configured,1) ,OTU(@2a0924d5@.Control.Stream.EnableSelected) OTU(@2a0924d5@.Control.Stream.DisableSelected) ] ] ,[OTU(@2a0924d5@.Control.Stream.SetSelectedToActive) ,COP(@5ad51bb9@[103+@24081be7@*2],@2321931e@,1) ,[XIC(@2321931e@.8) OTL(@e8982e82@.0) ,XIO(@2321931e@.8) OTU(@e8982e82@.0) ] ,[XIC(@2321931e@.9) OTL(@e8982e82@.1) ,XIO(@2321931e@.9) OTU(@e8982e82@.1) ] ,[XIC(@2321931e@.10) OTL(@e8982e82@.2) ,XIO(@2321931e@.10) OTU(@e8982e82@.2) ] ,[XIC(@2321931e@.11) OTL(@e8982e82@.3) ,XIO(@2321931e@.11) OTU(@e8982e82@.3) ] ,MVM(@2321931e@,16#000F,@5b185797@) ADD(@5b185797@,1,@2a0924d5@.Status.Stream.Active) ,COP(@e8982e82@,@2a0924d5@.Status.Stream.EnableAlarm,1) ] ,[XIC(@2a0924d5@.Control.ResetAccumulators.ResetAccumulator1) OTU(@2a0924d5@.Control.ResetAccumulators.ResetAccumulator1) OTU(@3f5c84fa@.Util.Buffer.MeterSignals[1+@24081be7@*2].4) ,XIC(@2a0924d5@.Control.ResetAccumulators.ResetAccumulator2) OTU(@2a0924d5@.Control.ResetAccumulators.ResetAccumulator2) OTU(@3f5c84fa@.Util.Buffer.MeterSignals[1+@24081be7@*2].5) ,XIC(@2a0924d5@.Control.ResetAccumulators.ResetAccumulator3) OTU(@2a0924d5@.Control.ResetAccumulators.ResetAccumulator3) OTU(@3f5c84fa@.Util.Buffer.MeterSignals[1+@24081be7@*2].6) ,XIC(@2a0924d5@.Control.ResetAccumulators.ResetAccumulator4) OTU(@2a0924d5@.Control.ResetAccumulators.ResetAccumulator4) OTU(@3f5c84fa@.Util.Buffer.MeterSignals[1+@24081be7@*2].7) ,XIC(@2a0924d5@.Archive.Write.Daily) OTU(@2a0924d5@.Archive.Write.Daily) OTU(@3f5c84fa@.Util.Buffer.MeterSignals[1+@24081be7@*2].8) ,XIC(@2a0924d5@.Archive.Write.Hourly) OTU(@2a0924d5@.Archive.Write.Hourly) OTU(@3f5c84fa@.Util.Buffer.MeterSignals[1+@24081be7@*2].9) ] ,OTU(@3f5c84fa@.Util.Block.InterruptPending.EnableDisable) OTL(@3f5c84fa@.Util.Block.InterruptComplete.EnableDisable) OTU(@3f5c84fa@.Util.Block.InterruptPending.Now) ];
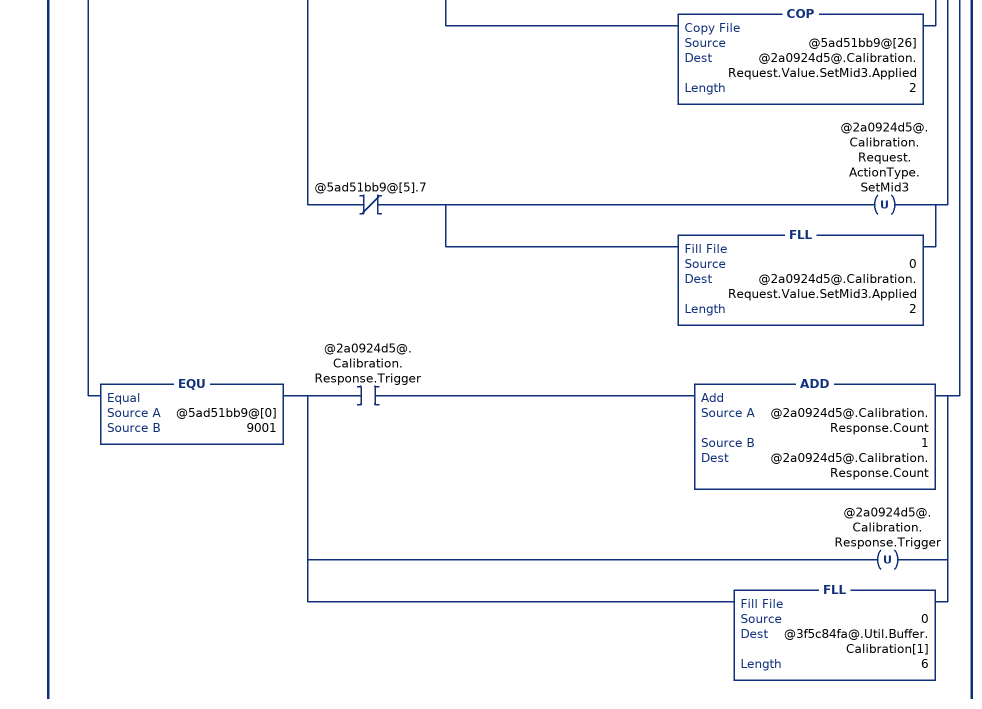
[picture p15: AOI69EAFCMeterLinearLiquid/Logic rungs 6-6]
   // Meter transmitter calibration.
   6: XIC(@2d889a89@)[EQU(@5ad51bb9@[0],9000) ,EQU(@5ad51bb9@[0],9001) ][MVM(@5ad51bb9@[3],16#0F00,@c9c083f8@) ,DIV(@c9c083f8@,16#100,@c9c083f8@) ]EQU(@c9c083f8@,@24081be7@)XIO(@5ad51bb9@[3].14)[EQU(@5ad51bb9@[0],9000) [XIO(@d5405e9b@) ADD(@2a0924d5@.Calibration.Request.Count,1,@2a0924d5@.Calibration.Request.Count) ,OTL(@d5405e9b@) [COP(@5ad51bb9@[3],@1d93410d@,1) ,MVM(@1d93410d@,16#000F,@4a4a3092@) ] ,[EQU(@4a4a3092@,0) [OTL(@2a0924d5@.Calibration.Request.ProcessVariable.PulseFrequency) ,OTU(@2a0924d5@.Calibration.Request.ProcessVariable.Temperature) ,OTU(@2a0924d5@.Calibration.Request.ProcessVariable.Pressure) ,OTU(@2a0924d5@.Calibration.Request.ProcessVariable.Density) ,OTU(@2a0924d5@.Calibration.Request.ProcessVariable.WaterContent) ] ,EQU(@4a4a3092@,1) [OTL(@2a0924d5@.Calibration.Request.ProcessVariable.Temperature) ,OTU(@2a0924d5@.Calibration.Request.ProcessVariable.PulseFrequency) ,OTU(@2a0924d5@.Calibration.Request.ProcessVariable.Pressure) ,OTU(@2a0924d5@.Calibration.Request.ProcessVariable.Density) ,OTU(@2a0924d5@.Calibration.Request.ProcessVariable.WaterContent) ] ,EQU(@4a4a3092@,2) [OTL(@2a0924d5@.Calibration.Request.ProcessVariable.Pressure) ,OTU(@2a0924d5@.Calibration.Request.ProcessVariable.PulseFrequency) ,OTU(@2a0924d5@.Calibration.Request.ProcessVariable.Temperature) ,OTU(@2a0924d5@.Calibration.Request.ProcessVariable.Density) ,OTU(@2a0924d5@.Calibration.Request.ProcessVariable.WaterContent) ] ,EQU(@4a4a3092@,3) [OTL(@2a0924d5@.Calibration.Request.ProcessVariable.Density) ,OTU(@2a0924d5@.Calibration.Request.ProcessVariable.PulseFrequency) ,OTU(@2a0924d5@.Calibration.Request.ProcessVariable.Temperature) ,OTU(@2a0924d5@.Calibration.Request.ProcessVariable.Pressure) ,OTU(@2a0924d5@.Calibration.Request.ProcessVariable.WaterContent) ] ,EQU(@4a4a3092@,4) [OTL(@2a0924d5@.Calibration.Request.ProcessVariable.WaterContent) ,OTU(@2a0924d5@.Calibration.Request.ProcessVariable.PulseFrequency) ,OTU(@2a0924d5@.Calibration.Request.ProcessVariable.Temperature) ,OTU(@2a0924d5@.Calibration.Request.ProcessVariable.Pressure) ,OTU(@2a0924d5@.Calibration.Request.ProcessVariable.Density) ] ] ,[[XIC(@5ad51bb9@[5].2) [OTL(@2a0924d5@.Calibration.Request.ActionType.ZeroShift) ,COP(@5ad51bb9@[6],@2a0924d5@.Calibration.Request.Value.ZeroShift.Applied,2) ] ,XIO(@5ad51bb9@[5].2) [OTU(@2a0924d5@.Calibration.Request.ActionType.ZeroShift) ,FLL(0,@2a0924d5@.Calibration.Request.Value.ZeroShift.Applied,2) ] ] ,[XIC(@5ad51bb9@[5].3) [OTL(@2a0924d5@.Calibration.Request.ActionType.SetZero) ,COP(@5ad51bb9@[10],@2a0924d5@.Calibration.Request.Value.SetZero.Applied,2) ] ,XIO(@5ad51bb9@[5].3) [OTU(@2a0924d5@.Calibration.Request.ActionType.SetZero) ,FLL(0,@2a0924d5@.Calibration.Request.Value.SetZero.Applied,2) ] ] ,[XIC(@5ad51bb9@[5].4) [OTL(@2a0924d5@.Calibration.Request.ActionType.SetSpan) ,COP(@5ad51bb9@[14],@2a0924d5@.Calibration.Request.Value.SetSpan.Applied,2) ] ,XIO(@5ad51bb9@[5].4) [OTU(@2a0924d5@.Calibration.Request.ActionType.SetSpan) ,FLL(0,@2a0924d5@.Calibration.Request.Value.SetSpan.Applied,2) ] ] ,[XIC(@5ad51bb9@[5].5) [OTL(@2a0924d5@.Calibration.Request.ActionType.SetMid1) ,COP(@5ad51bb9@[18],@2a0924d5@.Calibration.Request.Value.SetMid1.Applied,2) ] ,XIO(@5ad51bb9@[5].5) [OTU(@2a0924d5@.Calibration.Request.ActionType.SetMid1) ,FLL(0,@2a0924d5@.Calibration.Request.Value.SetMid1.Applied,2) ] ] ,[XIC(@5ad51bb9@[5].6) [OTL(@2a0924d5@.Calibration.Request.ActionType.SetMid2) ,COP(@5ad51bb9@[22],@2a0924d5@.Calibration.Request.Value.SetMid2.Applied,2) ] ,XIO(@5ad51bb9@[5].6) [OTU(@2a0924d5@.Calibration.Request.ActionType.SetMid2) ,FLL(0,@2a0924d5@.Calibration.Request.Value.SetMid2.Applied,2) ] ] ,[XIC(@5ad51bb9@[5].7) [OTL(@2a0924d5@.Calibration.Request.ActionType.SetMid3) ,COP(@5ad51bb9@[26],@2a0924d5@.Calibration.Request.Value.SetMid3.Applied,2) ] ,XIO(@5ad51bb9@[5].7) [OTU(@2a0924d5@.Calibration.Request.ActionType.SetMid3) ,FLL(0,@2a0924d5@.Calibration.Request.Value.SetMid3.Applied,2) ] ] ] ] ,EQU(@5ad51bb9@[0],9001) [XIC(@2a0924d5@.Calibration.Response.Trigger) ADD(@2a0924d5@.Calibration.Response.Count,1,@2a0924d5@.Calibration.Response.Count) ,OTU(@2a0924d5@.Calibration.Response.Trigger) ,FLL(0,@3f5c84fa@.Util.Buffer.Calibration[1],6) ] ];
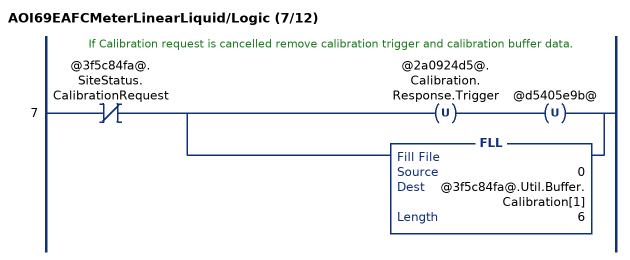
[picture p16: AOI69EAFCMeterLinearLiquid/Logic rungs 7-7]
   // If Calibration request is cancelled remove calibration trigger and calibration buffer data.
   7: XIO(@3f5c84fa@.SiteStatus.CalibrationRequest)[OTU(@2a0924d5@.Calibration.Response.Trigger) OTU(@d5405e9b@) ,FLL(0,@3f5c84fa@.Util.Buffer.Calibration[1],6) ];
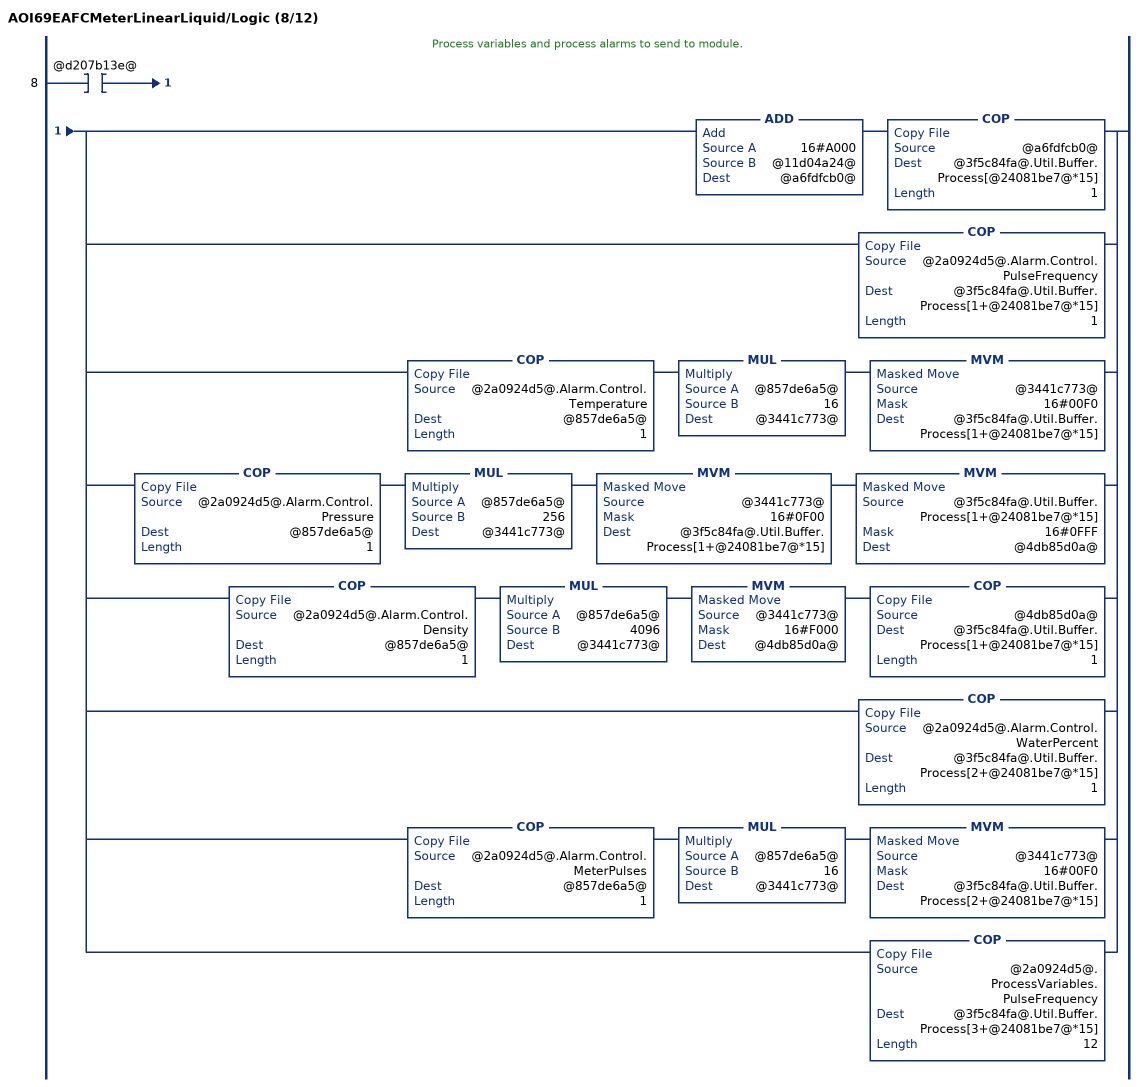
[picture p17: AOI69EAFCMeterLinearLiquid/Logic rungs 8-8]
   // Process variables and process alarms to send to module.
   8: XIC(@d207b13e@)[ADD(16#A000,@11d04a24@,@a6fdfcb0@) COP(@a6fdfcb0@,@3f5c84fa@.Util.Buffer.Process[@24081be7@*15],1) ,COP(@2a0924d5@.Alarm.Control.PulseFrequency,@3f5c84fa@.Util.Buffer.Process[1+@24081be7@*15],1) ,COP(@2a0924d5@.Alarm.Control.Temperature,@857de6a5@,1) MUL(@857de6a5@,16,@3441c773@) MVM(@3441c773@,16#00F0,@3f5c84fa@.Util.Buffer.Process[1+@24081be7@*15]) ,COP(@2a0924d5@.Alarm.Control.Pressure,@857de6a5@,1) MUL(@857de6a5@,256,@3441c773@) MVM(@3441c773@,16#0F00,@3f5c84fa@.Util.Buffer.Process[1+@24081be7@*15]) MVM(@3f5c84fa@.Util.Buffer.Process[1+@24081be7@*15],16#0FFF,@4db85d0a@) ,COP(@2a0924d5@.Alarm.Control.Density,@857de6a5@,1) MUL(@857de6a5@,4096,@3441c773@) MVM(@3441c773@,16#F000,@4db85d0a@) COP(@4db85d0a@,@3f5c84fa@.Util.Buffer.Process[1+@24081be7@*15],1) ,COP(@2a0924d5@.Alarm.Control.WaterPercent,@3f5c84fa@.Util.Buffer.Process[2+@24081be7@*15],1) ,COP(@2a0924d5@.Alarm.Control.MeterPulses,@857de6a5@,1) MUL(@857de6a5@,16,@3441c773@) MVM(@3441c773@,16#00F0,@3f5c84fa@.Util.Buffer.Process[2+@24081be7@*15]) ,COP(@2a0924d5@.ProcessVariables.PulseFrequency,@3f5c84fa@.Util.Buffer.Process[3+@24081be7@*15],12) ];
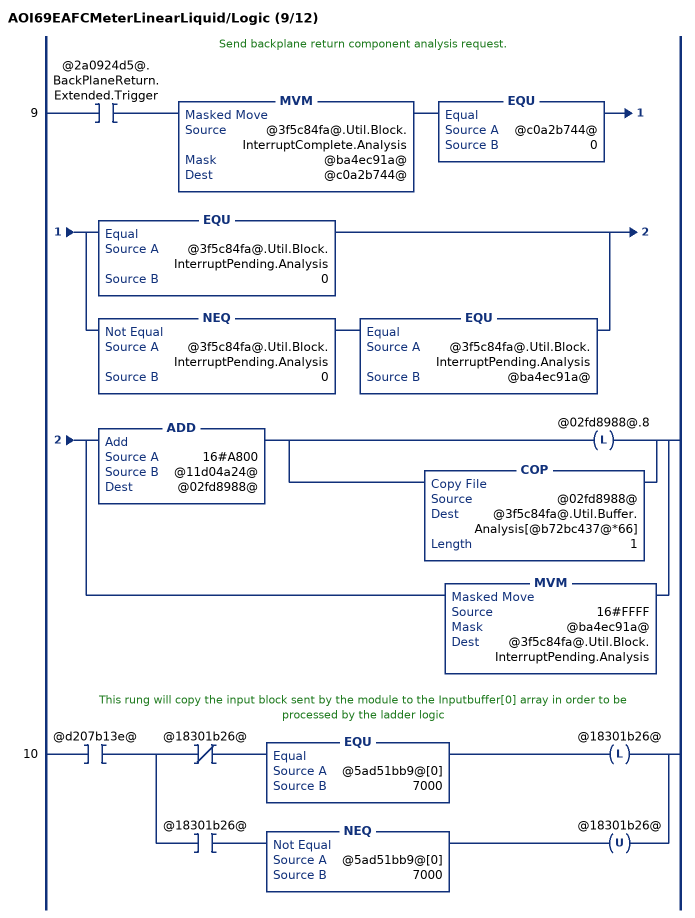
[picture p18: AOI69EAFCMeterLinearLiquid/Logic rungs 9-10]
   // Send backplane return component analysis request.
   9: XIC(@2a0924d5@.BackPlaneReturn.Extended.Trigger)MVM(@3f5c84fa@.Util.Block.InterruptComplete.Analysis,@ba4ec91a@,@c0a2b744@)EQU(@c0a2b744@,0)[EQU(@3f5c84fa@.Util.Block.InterruptPending.Analysis,0) ,NEQ(@3f5c84fa@.Util.Block.InterruptPending.Analysis,0) EQU(@3f5c84fa@.Util.Block.InterruptPending.Analysis,@ba4ec91a@) ][ADD(16#A800,@11d04a24@,@02fd8988@) [OTL(@02fd8988@.8) ,COP(@02fd8988@,@3f5c84fa@.Util.Buffer.Analysis[@b72bc437@*66],1) ] ,MVM(16#FFFF,@ba4ec91a@,@3f5c84fa@.Util.Block.InterruptPending.Analysis) ];
   // This rung will copy the input block sent by the module to the Inputbuffer[0] array in order to be processed by the ladder logic
   10: XIC(@d207b13e@)[XIO(@18301b26@) EQU(@5ad51bb9@[0],7000) OTL(@18301b26@) ,XIC(@18301b26@) NEQ(@5ad51bb9@[0],7000) OTU(@18301b26@) ];
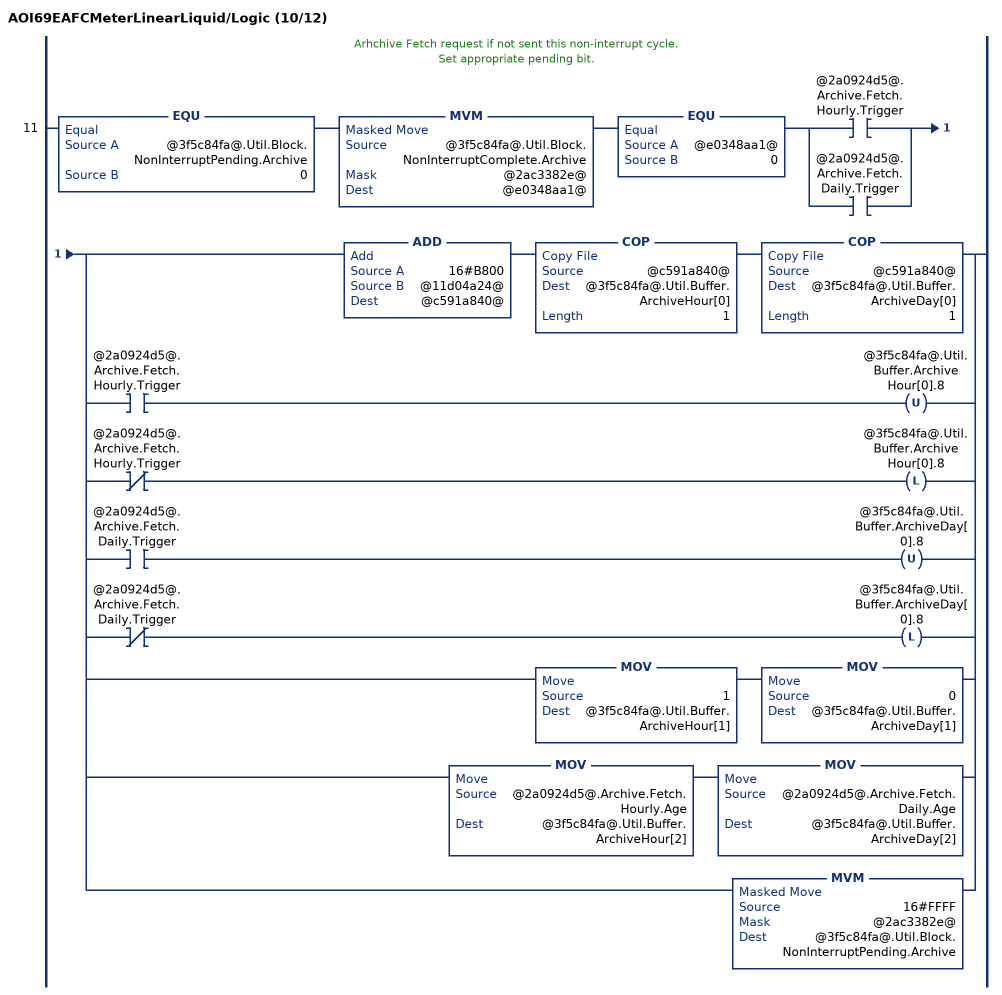
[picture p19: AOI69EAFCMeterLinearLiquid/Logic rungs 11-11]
   // Arhchive Fetch request if not sent this non-interrupt cycle.
   // Set appropriate pending bit.
   11: EQU(@3f5c84fa@.Util.Block.NonInterruptPending.Archive,0)MVM(@3f5c84fa@.Util.Block.NonInterruptComplete.Archive,@2ac3382e@,@e0348aa1@)EQU(@e0348aa1@,0)[XIC(@2a0924d5@.Archive.Fetch.Hourly.Trigger) ,XIC(@2a0924d5@.Archive.Fetch.Daily.Trigger) ][ADD(16#B800,@11d04a24@,@c591a840@) COP(@c591a840@,@3f5c84fa@.Util.Buffer.ArchiveHour[0],1) COP(@c591a840@,@3f5c84fa@.Util.Buffer.ArchiveDay[0],1) ,[XIC(@2a0924d5@.Archive.Fetch.Hourly.Trigger) OTU(@3f5c84fa@.Util.Buffer.ArchiveHour[0].8) ,XIO(@2a0924d5@.Archive.Fetch.Hourly.Trigger) OTL(@3f5c84fa@.Util.Buffer.ArchiveHour[0].8) ] ,[XIC(@2a0924d5@.Archive.Fetch.Daily.Trigger) OTU(@3f5c84fa@.Util.Buffer.ArchiveDay[0].8) ,XIO(@2a0924d5@.Archive.Fetch.Daily.Trigger) OTL(@3f5c84fa@.Util.Buffer.ArchiveDay[0].8) ] ,MOV(1,@3f5c84fa@.Util.Buffer.ArchiveHour[1]) MOV(0,@3f5c84fa@.Util.Buffer.ArchiveDay[1]) ,MOV(@2a0924d5@.Archive.Fetch.Hourly.Age,@3f5c84fa@.Util.Buffer.ArchiveHour[2]) MOV(@2a0924d5@.Archive.Fetch.Daily.Age,@3f5c84fa@.Util.Buffer.ArchiveDay[2]) ,MVM(16#FFFF,@2ac3382e@,@3f5c84fa@.Util.Block.NonInterruptPending.Archive) ];
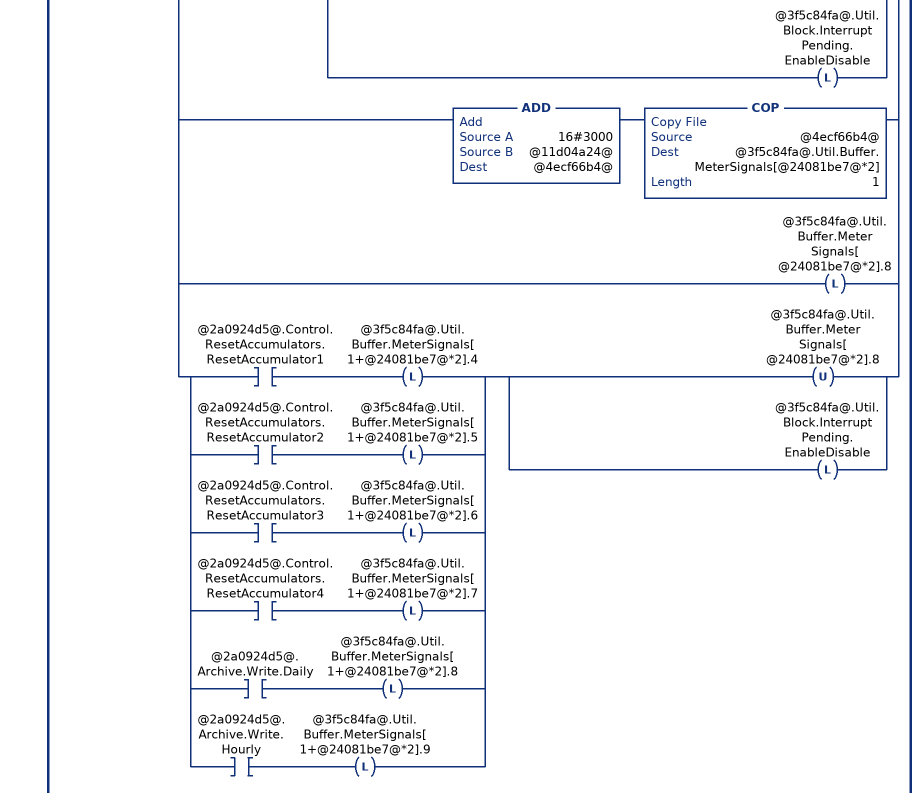
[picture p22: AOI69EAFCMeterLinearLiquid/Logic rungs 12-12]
   // Meter Enable.
   // Meter Disable.
   // Stream Select.
   // Stream Enable.
   // Stream Disable.
   // Set pending bit if not set this interrupt cycle.
   12: XIO(@3f5c84fa@.Util.Block.InterruptComplete.EnableDisable)[LIM(1,@2a0924d5@.Control.Stream.Selected,12) CPT(@f1f6e1ec@,2**(@2a0924d5@.Control.Stream.Selected-1)) ,[XIC(@2a0924d5@.Control.Meter.Enable) MVM(16#FFFF,@2ac3382e@,@3f5c84fa@.Util.Buffer.MeterEnableDisable[1]) MVM(16#0000,@2ac3382e@,@3f5c84fa@.Util.Buffer.MeterEnableDisable[3]) ,XIC(@2a0924d5@.Control.Meter.Disable) MVM(16#FFFF,@2ac3382e@,@3f5c84fa@.Util.Buffer.MeterEnableDisable[3]) MVM(16#0000,@2ac3382e@,@3f5c84fa@.Util.Buffer.MeterEnableDisable[1]) ] OTL(@3f5c84fa@.Util.Block.InterruptPending.EnableDisable) ,[ADD(16#CC00,@11d04a24@,@42febd3d@) COP(@42febd3d@,@3f5c84fa@.Util.Buffer.StreamEnable[@24081be7@*3],1) ,XIO(@2a0924d5@.Control.Stream.EnableSelected) OTL(@3f5c84fa@.Util.Buffer.StreamEnable[@24081be7@*3].8) ,XIC(@2a0924d5@.Control.Stream.EnableSelected) [OTU(@3f5c84fa@.Util.Buffer.StreamEnable[@24081be7@*3].8) ,COP(@f1f6e1ec@,@3f5c84fa@.Util.Buffer.StreamEnable[1+@24081be7@*3],1) ,OTL(@3f5c84fa@.Util.Block.InterruptPending.EnableDisable) ] ] ,[ADD(16#C800,@11d04a24@,@35bf0d3f@) COP(@35bf0d3f@,@3f5c84fa@.Util.Buffer.StreamDisable[@24081be7@*3],1) ,XIO(@2a0924d5@.Control.Stream.DisableSelected) OTL(@3f5c84fa@.Util.Buffer.StreamDisable[@24081be7@*3].8) ,XIC(@2a0924d5@.Control.Stream.DisableSelected) [OTU(@3f5c84fa@.Util.Buffer.StreamDisable[@24081be7@*3].8) ,COP(@f1f6e1ec@,@3f5c84fa@.Util.Buffer.StreamDisable[1+@24081be7@*3],1) ,OTL(@3f5c84fa@.Util.Block.InterruptPending.EnableDisable) ] ] ,[ADD(16#3C00,@11d04a24@,@e611f268@) COP(@e611f268@,@3f5c84fa@.Util.Buffer.StreamSelect[@24081be7@*2],1) ,XIO(@2a0924d5@.Control.Stream.SetSelectedToActive) OTL(@3f5c84fa@.Util.Buffer.StreamSelect[@24081be7@*2].8) ,XIC(@2a0924d5@.Control.Stream.SetSelectedToActive) [OTU(@3f5c84fa@.Util.Buffer.StreamSelect[@24081be7@*2].8) ,MOV(@2a0924d5@.Control.Stream.Selected,@3f5c84fa@.Util.Buffer.StreamSelect[1+@24081be7@*2]) ,OTL(@3f5c84fa@.Util.Block.InterruptPending.EnableDisable) ] ] ,[ADD(16#3000,@11d04a24@,@4ecf66b4@) COP(@4ecf66b4@,@3f5c84fa@.Util.Buffer.MeterSignals[@24081be7@*2],1) ,OTL(@3f5c84fa@.Util.Buffer.MeterSignals[@24081be7@*2].8) ,[XIC(@2a0924d5@.Control.ResetAccumulators.ResetAccumulator1) OTL(@3f5c84fa@.Util.Buffer.MeterSignals[1+@24081be7@*2].4) ,XIC(@2a0924d5@.Control.ResetAccumulators.ResetAccumulator2) OTL(@3f5c84fa@.Util.Buffer.MeterSignals[1+@24081be7@*2].5) ,XIC(@2a0924d5@.Control.ResetAccumulators.ResetAccumulator3) OTL(@3f5c84fa@.Util.Buffer.MeterSignals[1+@24081be7@*2].6) ,XIC(@2a0924d5@.Control.ResetAccumulators.ResetAccumulator4) OTL(@3f5c84fa@.Util.Buffer.MeterSignals[1+@24081be7@*2].7) ,XIC(@2a0924d5@.Archive.Write.Daily) OTL(@3f5c84fa@.Util.Buffer.MeterSignals[1+@24081be7@*2].8) ,XIC(@2a0924d5@.Archive.Write.Hourly) OTL(@3f5c84fa@.Util.Buffer.MeterSignals[1+@24081be7@*2].9) ] [OTU(@3f5c84fa@.Util.Buffer.MeterSignals[@24081be7@*2].8) ,OTL(@3f5c84fa@.Util.Block.InterruptPending.EnableDisable) ] ] ];
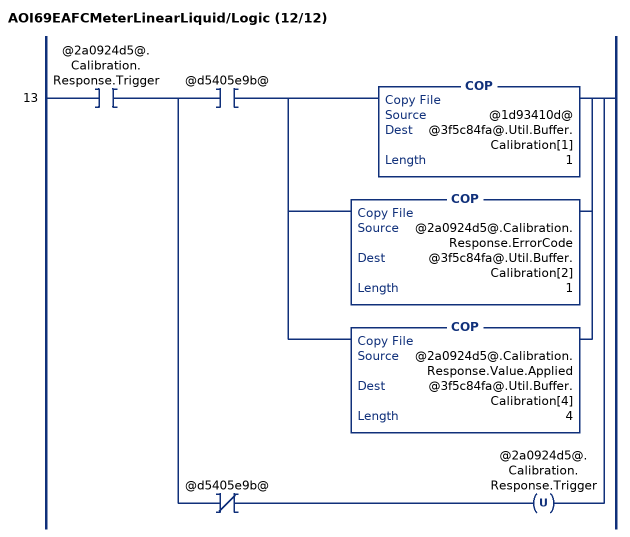
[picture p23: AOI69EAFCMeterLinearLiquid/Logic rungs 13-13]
   13: XIC(@2a0924d5@.Calibration.Response.Trigger)[XIC(@d5405e9b@) [COP(@1d93410d@,@3f5c84fa@.Util.Buffer.Calibration[1],1) ,COP(@2a0924d5@.Calibration.Response.ErrorCode,@3f5c84fa@.Util.Buffer.Calibration[2],1) ,COP(@2a0924d5@.Calibration.Response.Value.Applied,@3f5c84fa@.Util.Buffer.Calibration[4],4) ] ,XIO(@d5405e9b@) OTU(@2a0924d5@.Calibration.Response.Trigger) ];
END_ROUTINE

ROUTINE Prescan   (* ladder *)
// Prescan
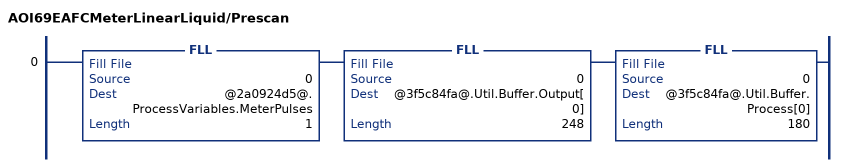
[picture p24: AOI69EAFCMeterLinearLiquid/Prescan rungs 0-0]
   0: FLL(0,@2a0924d5@.ProcessVariables.MeterPulses,1)FLL(0,@3f5c84fa@.Util.Buffer.Output[0],248)FLL(0,@3f5c84fa@.Util.Buffer.Process[0],180);
END_ROUTINE
END_ADD_ON_INSTRUCTION

VAR_GLOBAL   (* controller tags *)
   Local:1:I : AB:1756_MODULE_INT_496Bytes:I:0;
   AFC : AFCEModuleDef;
   AOI69EAFCMeter04LinearLiquid : AOI69EAFCMeterLinearLiquid;
   AFCMeter04LinearLiquid : AFCEMeterLinearLiquid;
END_VAR

PROGRAM MainProgram

ROUTINE MainRoutine   (* ladder *)
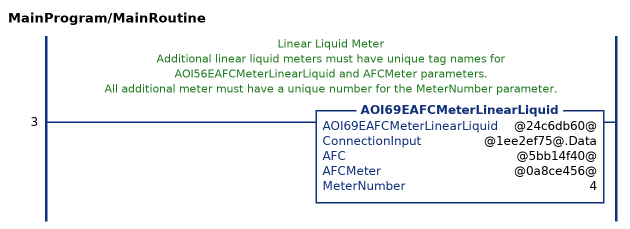
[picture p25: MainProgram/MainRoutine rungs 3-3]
   // Linear Liquid Meter
   // Additional linear liquid meters must have unique tag names for AOI56EAFCMeterLinearLiquid and AFCMeter parameters.
   // All additional meter must have a unique number for the MeterNumber parameter.
   3: AOI69EAFCMeterLinearLiquid(@24c6db60@,@1ee2ef75@.Data,@5bb14f40@,@0a8ce456@,4);
END_ROUTINE
END_PROGRAM
